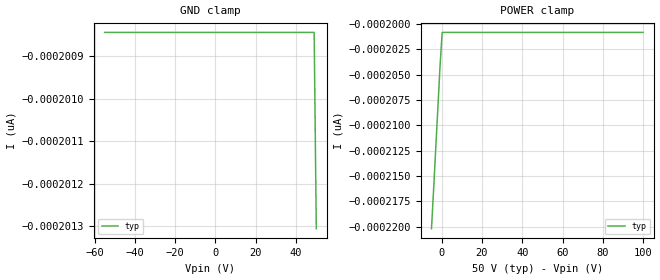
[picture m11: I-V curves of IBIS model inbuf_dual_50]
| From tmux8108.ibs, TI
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| inbuf_dual_50
[Model]   inbuf_dual_50
Model_type   Input
Vinl = 1.3
Vinh = 0.8
|   typ   min   max
C_comp   4.014581e-13   NA   NA
[Voltage Range]   50   NA   NA
[Temperature Range]   27   NA   NA
[Power Clamp Reference]   50   NA   NA
[GND Clamp Reference]   0   NA   NA
[GND Clamp]
|   Voltage   I(typ)   I(min)   I(max)
-55V      -200.8pA   NA         NA
-53.94V   -200.8pA   NA         NA
48.94V    -200.8pA   NA         NA
50V       -201.3pA   NA         NA
[POWER Clamp]
|   Voltage   I(typ)   I(min)   I(max)
-5V       -220.2pA   NA         NA
-3.939V   -216.3pA   NA         NA
-757.6mV  -204.2pA   NA         NA
303mV     -200.8pA   NA         NA
100V      -200.8pA   NA         NA
